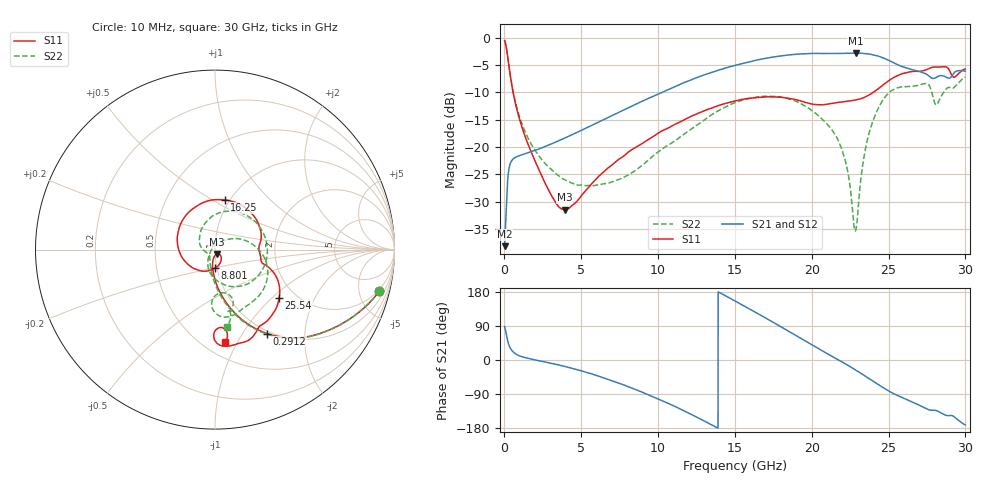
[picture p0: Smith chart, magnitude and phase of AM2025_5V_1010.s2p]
!Keysight Technologies,N5245B,MY58422270,A.16.20.02
!Date: Tuesday, July 14, 2026 01:08:33
!Correction: S11(C  2-Port  )
!S21(C  2-Port  )
!S12(C  2-Port  )
!S22(C  2-Port  )
!S2P File: Measurements: S11, S21, S12, S22:
# Hz S  dB  R 50
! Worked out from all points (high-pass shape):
!   3201 points, 10 MHz to 30 GHz, reference 50 ohm
!   highest |S21| = -2.81 dB at 22.85 GHz (marker M1); lowest = -38.1 dB at 10 MHz (marker M2)
!   |S21| within 3 dB of the highest: 14.07 GHz to 26.5 GHz (12.43 GHz wide, 61.3 % of centre)
!   lowest |S11| = -31.4 dB at 3.927 GHz (marker M3), VSWR 1.06, Z = 51 - j2.52 ohm
!   |S11| at or under -10 dB: 564.4 MHz to 23.99 GHz (23.42 GHz wide, 191 % of centre)
!   |S22| runs from -35.3 to -0.5 dB; largest |S21 - S12| = 0.0048
!   S11 on the Smith chart (normalised r, x): 10 MHz: 1.76, -7.56; 291.2 MHz: 0.96, -1.30; 8.801 GHz: 0.97, -0.21; 16.25 GHz: 0.95, +0.57; 25.54 GHz: 1.65, -1.11; 30 GHz: 0.64, -0.89
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1e7  -0.50 -14.3  -38.10 88.1  -35.45 95.2  -0.50 -14.1
2.911562e8  -5.17 -58.1  -24.00 39.6  -24.02 39.3  -5.15 -58.4
6.379156e8  -11.03 -79.8  -21.98 18.8  -22.03 18.3  -10.86 -80.4
1.537616e9  -19.48 -96.9  -21.02 4.2  -21.02 4.3  -18.36 -99.8
3.927444e9  -31.44 -67.4  -18.33 -17.1  -18.32 -17.1  -25.95 -125.6
5.014581e9  -28.85 -46.9  -16.91 -28.8  -16.91 -28.9  -26.92 -135.6
8.800819e9  -19.61 -91.2  -11.81 -82.2  -11.81 -82.3  -23.66 -178.9
1.000979e10  -17.43 -116.0  -10.28 -102.9  -10.28 -103.0  -20.86 159.9
1.245585e10  -14.00 -177.2  -7.36 -149.6  -7.36 -149.7  -16.10 111.0
1.5005e10  -11.59 112.3  -5.06 155.9  -5.06 155.9  -11.87 50.9
1.625146e10  -10.99 79.1  -4.19 128.1  -4.19 128.1  -10.94 19.5
1.817269e10  -10.94 34.2  -3.25 83.4  -3.25 83.4  -10.93 -28.1
2.000958e10  -12.12 5.3  -2.87 39.9  -2.87 39.9  -13.31 -69.7
2.187458e10  -11.78 -9.2  -2.87 -2.9  -2.87 -3.0  -19.76 -112.3
2.233381e10  -11.62 -12.8  -2.84 -13.6  -2.84 -13.7  -24.36 -127.8
2.284926e10  -11.39 -15.2  -2.81 -26.2  -2.82 -26.2  -35.30 136.1
2.367398e10  -10.55 -17.2  -2.96 -47.5  -2.96 -47.5  -18.03 29.4
2.500479e10  -7.87 -28.2  -4.12 -81.6  -4.12 -81.6  -10.11 -20.1
2.553899e10  -6.99 -37.0  -4.86 -92.8  -4.87 -92.8  -9.20 -38.1
2.749771e10  -5.79 -63.5  -6.70 -129.2  -6.70 -129.2  -8.39 -80.7
2.812562e10  -5.36 -73.7  -7.21 -133.7  -7.20 -133.8  -12.26 -80.2
3e10  -5.72 -83.6  -6.14 -171.2  -6.11 -171.4  -7.18 -81.2
